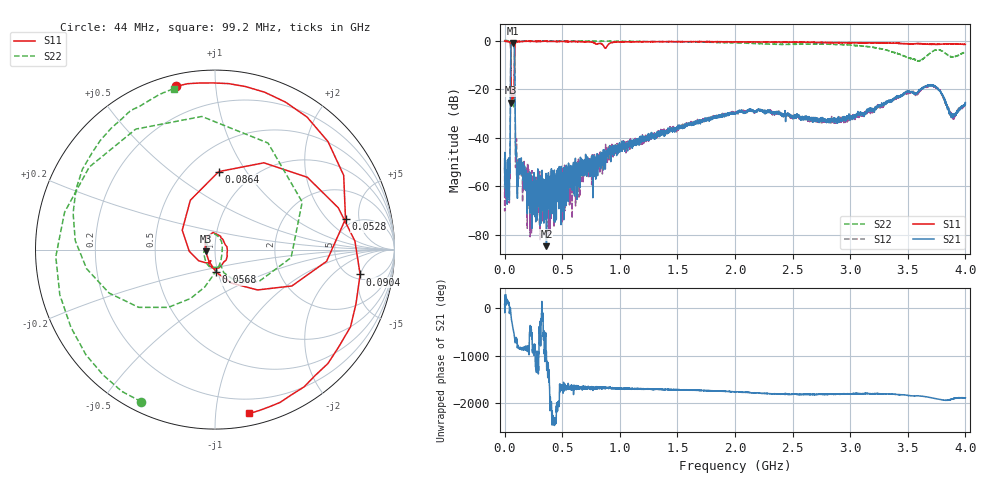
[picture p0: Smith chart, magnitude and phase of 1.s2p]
#  HZ  S  DB  R  50.00
! Rohde & Schwarz Vector Network Analyzer
! Rohde-Schwarz,ZNL6-2Port,1323001206101378,1.50.1.34-21.10.1.104
! Created: UTC 7/31/2023, 2:27:27 AM
! freq[Hz]  db:S11  ang:S11  db:S21  ang:S21  db:S12  ang:S12  db:S22  ang:S22
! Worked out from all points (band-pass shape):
!   5001 points, 5 kHz to 4 GHz, reference 50 ohm
!   highest |S21| = -1.01 dB at 68.8 MHz (marker M1); lowest = -84.6 dB at 363.2 MHz (marker M2)
!   |S21| within 3 dB of the highest: 54.27 MHz to 85.22 MHz (30.96 MHz wide, 44.4 % of centre)
!   lowest |S11| = -25.6 dB at 58.4 MHz (marker M3), VSWR 1.11, Z = 45.1 - j0.814 ohm
!   |S11| at or under -10 dB: 55.26 MHz to 85.67 MHz (30.41 MHz wide, 43.2 % of centre)
!   |S22| runs from -27.3 to 0.0 dB; largest |S21 - S12| = 0.019
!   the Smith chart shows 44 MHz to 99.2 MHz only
!   S11 on the Smith chart (normalised r, x): 44 MHz: 0.05, +0.79; 52.8 MHz: 4.27, +3.30; 56.8 MHz: 0.98, -0.25; 86.4 MHz: 0.71, +0.76; 90.4 MHz: 5.85, -4.97; 99.2 MHz: 0.09, -1.23
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5000  -0.21 -179.9  -52.73 84.2  -52.30 -64.4  -0.01 0.2
2.720497e7  -0.39 148.0  -57.79 123.6  -52.26 164.3  -0.07 -42.9
4.400494e7  -0.58 103.6  -53.01 -104.3  -51.85 -83.9  -0.52 -115.8
5.280493e7  -2.53 13.2  -8.46 -65.0  -8.49 -65.1  -3.57 63.5
5.680493e7  -17.96 -86.9  -1.58 173.5  -1.66 173.4  -17.22 -69.1
5.840493e7  -25.55 -170.2  -1.35 139.9  -1.33 140.6  -20.75 -68.3
6.880491e7  -23.31 13.0  -1.01 -4.1  -1.09 -3.8  -25.74 156.8
8.640489e7  -7.23 87.3  -6.19 84.7  -6.15 84.2  -5.46 -142.9
9.040489e7  -1.72 -9.7  -21.60 6.7  -21.59 6.6  -1.47 156.6
9.920488e7  -0.60 -78.1  -45.04 106.4  -43.86 94.0  -0.67 104.3
1.112049e8  -0.44 -110.6  -64.90 -88.9  -57.73 -72.6  -0.42 75.6
1.240048e8  -0.39 -127.1  -49.10 -126.1  -51.42 -121.3  -0.35 59.2
2.408047e8  -0.32 -165.5  -67.77 -59.8  -64.34 -82.7  -0.19 18.1
3.632045e8  -0.26 -174.1  -84.58 81.7  -61.41 132.0  -0.15 7.0
6.672042e8  -0.51 167.6  -52.54 116.4  -55.30 103.0  -0.18 -7.3
1.333603e9  -0.42 160.6  -39.32 100.2  -39.50 93.5  -0.44 -30.3
2.000002e9  -0.56 151.8  -30.22 45.0  -29.64 42.6  -0.98 -53.4
2.667202e9  -0.74 147.7  -31.74 -10.7  -32.95 -11.4  -1.46 -71.9
3.333601e9  -1.06 144.1  -24.98 -3.5  -25.06 -2.6  -4.21 -97.1
3.704e9  -1.52 140.5  -18.23 -82.7  -18.80 -79.9  -4.87 -61.7
3.8856e9  -1.38 138.5  -30.80 -111.6  -31.17 -104.4  -6.77 -69.5
4e9  -1.56 135.5  -25.53 -84.4  -26.46 -75.4  -4.66 -55.1
